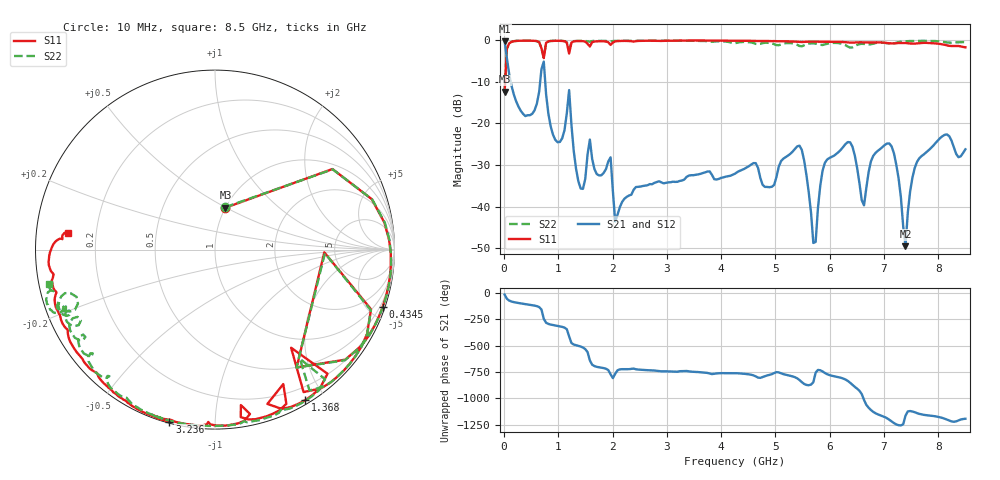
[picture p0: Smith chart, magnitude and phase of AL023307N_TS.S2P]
!AVX CORPORATION
!PN: AL023307_TS
!DESCRIPTION: AIR CORE INDUCTOR, 307nH, 16 turns
!Agilent Technologies,E5071C,MY46102230,A.09.54
!Date: Mon Sep 03 16:47:51 2012
!Data & Calibration Information:
!Freq	S11:SOLT2(ON)	S21:SOLT2(ON)	S12:SOLT2(ON)	S22:SOLT2(ON)
# Hz S dB R 50
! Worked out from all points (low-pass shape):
!   201 points, 10 MHz to 8.5 GHz, reference 50 ohm
!   highest |S21| = -0.23 dB at 10 MHz (marker M1); lowest = -49.5 dB at 7.396 GHz (marker M2)
!   |S21| within 3 dB of the highest: start of sweep to 40.83 MHz
!   lowest |S11| = -12.4 dB at 10 MHz (marker M3), VSWR 1.63, Z = 50 + j24.8 ohm
!   |S11| at or under -10 dB: start of sweep to 19.74 MHz
!   |S22| runs from -12.3 to -0.1 dB; largest |S21 - S12| = 0.006
!   S11 on the Smith chart (normalised r, x): 10 MHz: 1.00, +0.50; 434.5 MHz: 0.24, -6.00; 1.368 GHz: 0.05, -1.77; 3.236 GHz: 0.01, -0.77; 8.5 GHz: 0.10, +0.06
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1e7  -12.38 76.0  -0.23 -14.5  -0.19 -14.7  -12.28 76.5
9.49e7  -0.75 17.8  -8.19 -71.9  -8.18 -72.0  -0.73 17.7
4.345e8  -0.11 -18.9  -18.03 -108.5  -18.03 -108.6  -0.10 -19.1
6.892e8  -1.95 -55.3  -6.93 -156.9  -6.92 -157.0  -1.95 -55.4
7.3165e8  -4.30 -1.4  -5.14 115.2  -5.13 115.2  -4.26 -1.9
9.439e8  -0.14 -40.4  -23.96 51.7  -23.96 51.6  -0.13 -40.4
1.1986e9  -3.20 -52.2  -11.99 -51.1  -11.99 -51.2  -2.27 -52.1
1.3684e9  -0.19 -59.0  -33.89 -141.5  -34.01 -141.5  -0.17 -58.8
1.4533e9  -0.23 -64.2  -35.75 -157.3  -35.79 -157.3  -0.17 -62.9
1.58065e9  -1.51 -63.1  -23.89 80.9  -23.88 81.0  -0.36 -67.0
2.0476e9  -0.28 -80.3  -43.57 -46.5  -43.82 -47.1  -0.16 -82.8
2.85415e9  -0.16 -103.9  -33.92 -20.3  -33.96 -20.1  -0.12 -102.9
3.2362e9  -0.06 -104.8  -33.84 -22.0  -33.77 -22.0  -0.13 -107.3
4.255e9  -0.10 -115.2  -32.10 -40.4  -32.09 -40.4  -0.74 -129.8
5.4436e9  -0.43 -133.6  -25.36 -105.9  -25.39 -106.0  -1.38 -153.9
5.6983e9  -0.34 -137.7  -48.75 -126.5  -48.28 -124.8  -0.76 -155.4
5.953e9  -0.37 -142.8  -28.69 -50.3  -28.71 -50.3  -0.87 -155.9
6.6322e9  -0.51 -155.6  -39.72 65.3  -39.83 64.8  -0.90 -159.4
7.09915e9  -0.73 -164.6  -24.84 -123.1  -24.86 -123.2  -0.85 -160.5
7.3963e9  -0.67 -169.3  -49.53 -84.3  -49.78 -81.2  -0.25 -159.6
7.60855e9  -0.77 -171.9  -29.26 -59.7  -29.22 -59.8  -0.16 -161.4
8.5e9  -1.70 173.4  -26.24 -113.2  -26.26 -113.3  -0.50 -168.1
